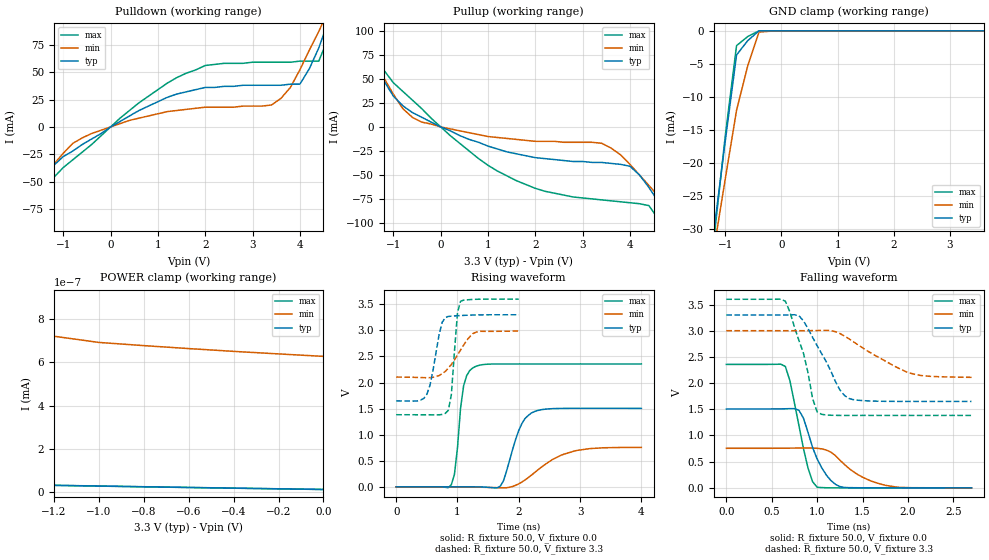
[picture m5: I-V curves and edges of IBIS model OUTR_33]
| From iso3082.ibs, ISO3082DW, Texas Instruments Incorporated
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[Model]   OUTR_33
Model_type   3-state
| Signals   R
Vmeas = 1.6V   |Reference voltage for timing measurements
Cref = 15pF   |Timing specification test load capacitance value
Vref = 0   |Timing specification test load voltage; GND
| variable   typ   min   max
C_comp   2.1pF   1.7pF   2.5pF
|   typ   min   max
[Temperature Range]   25.0   -40   125
[Voltage range]   3.3V   3.0V   3.6V
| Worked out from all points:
|   slope of the pulldown table from 0 to 0.495 V, typ, clamps not added: 40 ohm
|   slope of the pullup table from 0 to 0.495 V, typ, clamps not added: 45.4 ohm
|   GND clamp passes 1 mA (typ) near -0.54 V on its own axis
|   POWER clamp passes 1 mA (typ) near -2.27 V on its own axis
|   rising waveform, R_fixture 50.0, V_fixture 0.0: 20-80 % time 247ps typ, 564ps min, 121ps max; typ from 0 V to 1.5 V
|   falling waveform, R_fixture 50.0, V_fixture 0.0: 20-80 % time 208ps typ, 358ps min, 168ps max; typ from 1.5 V to 0 V
|   rising waveform, R_fixture 50.0, V_fixture 3.3: 20-80 % time 154ps typ, 299ps min, 84.2ps max; typ from 1.65 V to 3.3 V
|   falling waveform, R_fixture 50.0, V_fixture 3.3: 20-80 % time 296ps typ, 522ps min, 202ps max; typ from 3.3 V to 1.65 V
[Pulldown]
|   Voltage  I(typ)   I(min)   I(max)
-3.6V     -213mA     -167mA     -286mA
-2.2V     -106mA     -89mA      -137mA
-1.8V     -76mA      -66mA      -95mA
-1.2V     -35mA      -34mA      -46mA
-600mV    -16mA      -10mA      -23mA
2V        36mA       18mA       56mA
3.4V      38mA       20mA       59mA
4V        39mA       52mA       60mA
4.4V      72mA       87mA       60mA
4.6V      96mA       106mA      81mA
4.8V      120mA      124mA      106mA
7.5V      465mA      379mA      575mA
[Pullup]
|   Voltage   I(typ)  I(min)  I(max)
| Note that the[Pullup]voltage table is referenced to Vcc
| and is calculated using Vtable=Vcc - Vmeasured.
-3.6V     345mA      272mA      457mA
-2V       144mA      123mA      182mA
-1.5V     83mA       78mA       100mA
-1.2V     48mA       51mA       59mA
-600mV    15mA       10mA       28mA
800mV     -16mA      -8mA       -33mA
2V        -32mA      -15mA      -64mA
3.4V      -37mA      -17mA      -76mA
4V        -41mA      -39mA      -79mA
4.4V      -63mA      -61mA      -82mA
5V        -108mA     -95mA      -134mA
7.2V      -281mA     -221mA     -373mA
[GND_clamp]
|   Voltage   I(typ)   I(min)   I(max)
| Outputs in High Impedance (off)
-3.6V     -213mA     -167.2mA   -285.4mA
-1.2V     -30.16mA   -32.94mA   -31.43mA
-1.1V     -23.41mA   -27.68mA   -23.65mA
-1V       -16.66mA   -22.42mA   -15.87mA
-800mV    -3.66mA    -12.05mA   -2.249mA
-600mV    -1.479mA   -5.279mA   -861.1uA
-400mV    -1.657uA   -187.7uA   -4.797uA
0V        -40.79pA   -10.95nA   -39.6pA
3.6V      17.57pA    663pA      12.68pA
[POWER_clamp]
|   Voltage  I(typ)   I(min)   I(max)
| Note that the [POWER_clamp] voltage table is referenced to Vcc
| and is calculated using Vtable = Vcc - Vmeasured.
| Outputs in Tri-state.
-3.6V     130.9mA    132.2mA    129.3mA
-2.2V     594.7uA    10.13mA    942.3pA
-2.1V     8.158nA    6.126mA    495.1pA
-2V       5.434nA    2.119mA    47.98pA
-1.8V     1.376nA    388.9uA    43.35pA
-1.7V     41.24pA    194.6uA    41.32pA
-1.5V     37.53pA    132.3nA    37.35pA
-1.4V     35.76pA    755.1pA    35.42pA
-1.2V     32.25pA    720.1pA    31.79pA
-1V       28.85pA    691.4pA    28.37pA
-400mV    19.15pA    650.1pA    18.72pA
0V        12.94pA    627pA      12.68pA
[Ramp]
|   typ   min   max
dV/dt_r   0.903V/4.9ns   0.459V/11.3ns   1.414V/2.3ns
dV/dt_f   0.903V/4.0ns   0.459V/7.1ns   1.414V/3.3ns
R_load = 50
[Rising Waveform]
R_fixture = 50.0
V_fixture = 0.0
C_fixture = 0p
L_fixture = 0n
|   V(typ)   V(min)   V(max)
0s        489.7pV    12.09nV    431.9pV
900ps     17.01uV    282.3uV    42.76mV
950ps     27.86uV    217.4uV    238.3mV
1.1ns     89.93uV    -788.4uV   1.94V
1.3ns     -99.63uV   -4.419mV   2.312V
1.7ns     15.91mV    -17.3mV    2.357V
2ns       1.083V     58.82mV    2.357V
2.25ns    1.441V     266mV      2.357V
2.95ns    1.506V     698.7mV    2.357V
4ns       1.505V     756mV      2.357V
[Falling Waveform]
R_fixture = 50.0
V_fixture = 0.0
C_fixture = 0p
L_fixture = 0n
|   V(typ)   V(min)   V(max)
0s        1.505V     755.2mV    2.357V
650ps     1.51V      757.4mV    2.318V
700ps     1.512V     758.3mV    2.047V
800ps     1.481V     760.6mV    1.187V
900ps     1.057V     762mV      375.6mV
1ns       553.1mV    755.1mV    12.03mV
1.15ns    143.1mV    683mV      796.9uV
1.3ns     7.515mV    447.7mV    36.71uV
1.75ns    197.3uV    48.97mV    -2.819uV
2.7ns     -4.04uV    324.3uV    303.2nV
[Rising Waveform]
R_fixture = 50.0
V_fixture = 3.3
V_fixture_min = 3.0
V_fixture_max = 3.6
C_fixture = 0p
L_fixture = 0n
|   V(typ)   V(min)  V(max)
0s        1.649V     2.106V     1.383V
500ps     1.774V     2.093V     1.382V
550ps     1.943V     2.094V     1.382V
750ps     3.156V     2.171V     1.389V
850ps     3.268V     2.277V     1.468V
900ps     3.274V     2.348V     1.768V
1ns       3.282V     2.527V     3.341V
1.05ns    3.285V     2.625V     3.559V
1.3ns     3.296V     2.964V     3.597V
2ns       3.3V       2.989V     3.6V
[Falling Waveform]
R_fixture = 50.0
V_fixture = 3.3
V_fixture_min = 3.0
V_fixture_max = 3.6
C_fixture = 0p
L_fixture = 0n
|   V(typ)   V(min)  V(max)
0s        3.3V       3V         3.6V
650ps     3.3V       3V         3.563V
800ps     3.286V     3V         2.812V
850ps     3.187V     3V         2.569V
950ps     2.874V     3.002V     1.705V
1.05ns    2.561V     3.006V     1.404V
1.25ns    1.872V     2.947V     1.383V
1.35ns    1.707V     2.846V     1.383V
2ns       1.65V      2.201V     1.383V
2.7ns     1.65V      2.11V      1.383V
